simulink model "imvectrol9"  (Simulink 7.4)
settings: Solver=ode45  StartTime=0  StopTime=7  MaxStep=1e-3  RelTol=1e-4  AbsTol=1e-3
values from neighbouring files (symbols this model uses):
  Lm = eval(get(hLm,'String'))    [im3d.m]    (also in IMabc2.m = 4.5; imabcparam.m = 0.0847; IMabcrun0.m = 0.0847; IMabcrun1.m = 0.0847)
  Lr = Lrl+Lm    (= 4.6)    [IMabc2.m]    (also in IMabcf0.m = Lrl+Lm1; IMabcf1.m = Lrl+Lm1; imabcparam.m = 0.0589666666667; IMcur0.m)
  Lrl = eval(get(hLr,'String'))    [im3d.m]    (also in IMabc2.m = 0.1; imabcparam.m = 0.0025; IMabcrun0.m = 0.0025; IMabcrun1.m = 0.0025)
  Ls = Lsl+Lm    (= 4.6)    [IMabc2.m]    (also in IMabcf0.m = Lsl+Lm1; IMabcf1.m = Lsl+Lm1; imabcparam.m = 0.0589666666667; IMcur0.m)
  Lsl = eval(get(hLs,'String'))    [im3d.m]    (also in IMabc2.m = 0.1; imabcparam.m = 0.0025; IMabcrun0.m = 0.0025; IMabcrun1.m = 0.0025)
  Rr = input('Rotor resistance)[default = 2] =')    [Actac.m]    (also in im1phase.m = 0.3; im3d.m = eval(get(hRr,'String')); IMabc2.m = 0.02; imabcparam.m = 0.408)
  Rs = eval(get(hRs,'String'))    [im3d.m]    (also in IMabc2.m = 0.01; imabcparam.m = 0.531; IMabcrun0.m = 0.531; IMabcrun1.m = 0.531)
  wo = 2*pi*freq0    [calc0.m]    (also in IMabc2.m = 376.991118431; imabcparam.m = 376.991118431; IMabcrun0.m = 376.991118431; IMabcrun1.m = 376.991118431)
undefined symbols (not defined in the file or in its folder): fro, Lsp, Tr

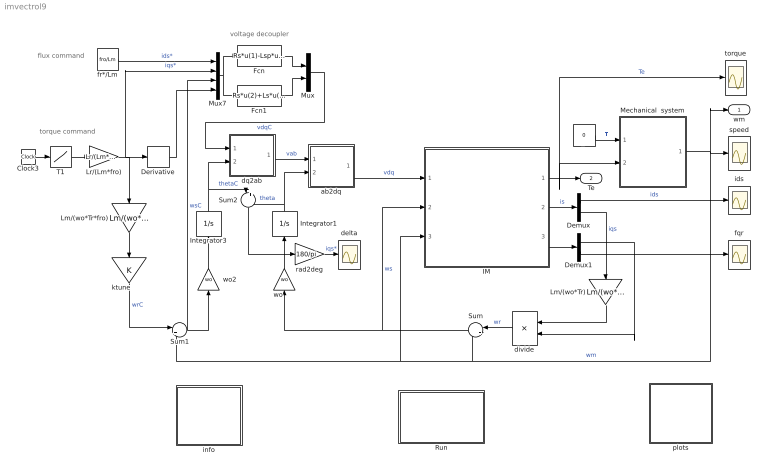
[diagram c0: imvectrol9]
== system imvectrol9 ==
  note: torque command
  note: flux command
  note: voltage decoupler
  Clock3 : Clock
  Demux : Demux  Outputs=2
  Demux1 : Demux  Outputs=2
  Derivative : Derivative
  Fcn : Fcn  Expr=Rs*u(1)-Lsp*u(2)*u(3)
  Fcn1 : Fcn  Expr=Rs*u(2)+Ls*u(1)*u(3)+Lsp*u(4)/wo
  IM : Subsystem
  Integrator1 : Integrator
  Integrator3 : Integrator
  Lm/(wo*Tr) : Gain  Gain=Lm/(wo*Tr)  ParameterDataType=sfix(16)  ParameterScaling=2^0  OutDataType=sfix(16)  OutScaling=2^0
  Lm/(wo*Tr*fro) : Gain  Gain=Lm/(wo*Tr*fro)  ParameterDataType=sfix(16)  ParameterScaling=2^0  OutDataType=sfix(16)  OutScaling=2^0
  Lr/(Lm*fro) : Gain  Gain=Lr/(Lm*fro)  ParameterDataType=sfix(16)  ParameterScaling=2^0  OutDataType=sfix(16)  OutScaling=2^0
  Mechanical  system : Subsystem  mask{H=0.3, Bm=1e-5}
      mask prompts: H "Inertia constant [s]"; Bm "Torque-speed coefficient"
  Mux : Mux  Inputs=2
  Mux7 : Mux
  Run : Subsystem
  Sum : Sum  Inputs=|++  OutDataType=sfix(16)  OutScaling=2^0
  Sum1 : Sum  Inputs=|++  OutDataType=sfix(16)  OutScaling=2^0
  Sum2 : Sum  Inputs=|+-  OutDataType=sfix(16)  OutScaling=2^0
  T1 : Lookup  InputValues=[0 1 1.5 2.5 3.5 4.5 5 8]  Table=[0 0 1 1 -1 -1 0 0]  OutDataType=sfix(16)  OutScaling=2^0
  Tl : Constant  Value=0  OutDataType=sfix(16)  OutScaling=2^0
  ab2dq : Subsystem
  delta : Scope
  divide : Product  Inputs=*/  OutDataType=sfix(16)  OutScaling=2^0
  dq2ab : Subsystem
  fqr : Scope
  fr*/Lm : Constant  Value=fro/Lm  OutDataType=sfix(16)  OutScaling=2^0
  ids : Scope
  info : Subsystem
  ktune : Gain  ParameterDataType=sfix(16)  ParameterScaling=2^0  OutDataType=sfix(16)  OutScaling=2^0
  plots : Subsystem
  rad2deg : Gain  Gain=180/pi  ParameterDataType=sfix(16)  ParameterScaling=2^0  OutDataType=sfix(16)  OutScaling=2^0
  speed : Scope
  torque : Scope
  wo : Gain  Gain=wo  ParameterDataType=sfix(16)  ParameterScaling=2^0  OutDataType=sfix(16)  OutScaling=2^0
  wo2 : Gain  Gain=wo  ParameterDataType=sfix(16)  ParameterScaling=2^0  OutDataType=sfix(16)  OutScaling=2^0
  wm : Outport
  Te : Outport  Port=2
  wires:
  Tl/1 -> Mechanical  system/1(Tl)  "Tl"
  Mechanical  system/1(wm) -> speed/1, Sum/2, IM/3(wm), Sum1/2, wm/1  "wm"
  IM/3(fr) -> Demux1/1
  Demux/2 -> Lm/(wo*Tr)/1  "iqs"
  Sum/1 -> IM/2(Iwk), wo/1  "ws"
  wo/1 -> Integrator1/1
  wo2/1 -> Integrator3/1
  Sum1/1 -> wo2/1, Mux7/3  "wsC"
  IM/1(Te) -> Mechanical  system/2(Te), torque/1, Te/1  "Te"
  Lm/(wo*Tr)/1 -> divide/1
  divide/1 -> Sum/1  "wr"
  dq2ab/1(ab) -> ab2dq/1(ab)  "vab"
  Fcn/1 -> Mux/1
  Mux/1 -> dq2ab/1(dq)  "vdqC"
  Mux7/1 -> Fcn/1, Fcn1/1
  Fcn1/1 -> Mux/2
  fr*/Lm/1 -> Mux7/1  "ids*"
  Lm/(wo*Tr*fro)/1 -> ktune/1
  Lr/(Lm*fro)/1 -> Mux7/2, Lm/(wo*Tr*fro)/1, Derivative/1  "iqs*"
  ktune/1 -> Sum1/1  "wrC"
  Clock3/1 -> T1/1
  T1/1 -> Lr/(Lm*fro)/1
  Derivative/1 -> Mux7/4
  Demux1/2 -> fqr/1
  ab2dq/1(dq) -> IM/1(vs)  "vdq"
  Demux/1 -> ids/1  "ids"
  Demux1/1 -> divide/2
  Integrator3/1 -> dq2ab/2(theta), Sum2/1  "thetaC"
  Integrator1/1 -> ab2dq/2(theta), Sum2/2  "theta"
  IM/2(is) -> Demux/1  "is"
  Sum2/1 -> rad2deg/1
  rad2deg/1 -> delta/1  "iqs*"

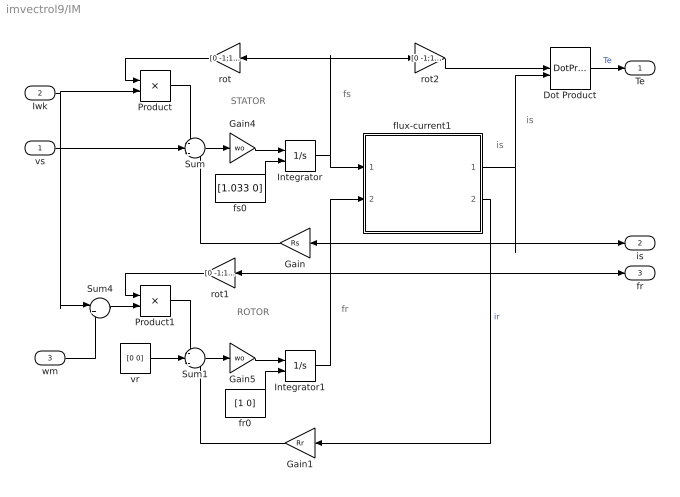
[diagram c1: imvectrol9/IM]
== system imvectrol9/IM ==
  note: ROTOR
  note: STATOR
  note: fs
  note: fr
  note: is
  note: is
  vs : Inport  OutDataType=sfix(16)  OutScaling=2^0
  Iwk : Inport  Port=2  OutDataType=sfix(16)  OutScaling=2^0
  wm : Inport  Port=3  OutDataType=sfix(16)  OutScaling=2^0
  Dot Product : DotProduct  OutDataType=fixdt(1, 16)  OutScaling=2^-10
  Gain : Gain  Gain=Rs  ParameterDataType=sfix(16)  ParameterScaling=2^0  OutDataType=sfix(16)  OutScaling=2^0
  Gain1 : Gain  Gain=Rr  ParameterDataType=sfix(16)  ParameterScaling=2^0  OutDataType=sfix(16)  OutScaling=2^0
  Gain4 : Gain  Gain=wo  ParameterDataType=sfix(16)  ParameterScaling=2^0  OutDataType=sfix(16)  OutScaling=2^0
  Gain5 : Gain  Gain=wo  ParameterDataType=sfix(16)  ParameterScaling=2^0  OutDataType=sfix(16)  OutScaling=2^0
  Integrator : Integrator  InitialConditionSource=external  InitialCondition=[1 0]
  Integrator1 : Integrator  InitialConditionSource=external  InitialCondition=[1 0]
  Product : Product  OutDataType=sfix(16)  OutScaling=2^0
  Product1 : Product  OutDataType=sfix(16)  OutScaling=2^0
  Sum : Sum  Inputs=-+-  OutDataType=sfix(16)  OutScaling=2^0
  Sum1 : Sum  Inputs=-+-  OutDataType=sfix(16)  OutScaling=2^0
  Sum4 : Sum  Inputs=|+-  OutDataType=sfix(16)  OutScaling=2^0
  flux-current1 : Subsystem
  fr0 : Constant  Value=[1 0]  OutDataType=sfix(16)  OutScaling=2^0
  fs0 : Constant  Value=[1.033 0]  OutDataType=sfix(16)  OutScaling=2^0
  rot : Gain  Gain=[0 -1;1 0]  Multiplication=Matrix(K*u)  ParameterDataType=sfix(16)  ParameterScaling=2^0  OutDataType=sfix(16)  OutScaling=2^0
  rot1 : Gain  Gain=[0 -1;1 0]  Multiplication=Matrix(K*u)  ParameterDataType=sfix(16)  ParameterScaling=2^0  OutDataType=sfix(16)  OutScaling=2^0
  rot2 : Gain  Gain=[0 -1;1 0]  Multiplication=Matrix(K*u)  ParameterDataType=sfix(16)  ParameterScaling=2^0  OutDataType=sfix(16)  OutScaling=2^0
  vr : Constant  Value=[0 0]  OutDataType=sfix(16)  OutScaling=2^0
  Te : Outport
  is : Outport  Port=2
  fr : Outport  Port=3
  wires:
  Gain/1 -> Sum/3
  vr/1 -> Sum1/2
  Integrator/1 -> flux-current1/1(fs), rot/1, rot2/1
  Integrator1/1 -> flux-current1/2(fr), rot1/1, fr/1
  Product1/1 -> Sum1/1
  rot1/1 -> Product1/1
  Product/1 -> Sum/1
  rot/1 -> Product/1
  rot2/1 -> Dot Product/1
  Sum4/1 -> Product1/2
  Sum/1 -> Gain4/1
  Gain4/1 -> Integrator/1
  Sum1/1 -> Gain5/1
  Gain5/1 -> Integrator1/1
  Dot Product/1 -> Te/1  "Te"
  vs/1 -> Sum/2
  Iwk/1 -> Product/2, Sum4/1
  wm/1 -> Sum4/2
  flux-current1/1(is) -> Gain/1, is/1, Dot Product/2
  fr0/1 -> Integrator1/2
  fs0/1 -> Integrator/2
  Gain1/1 -> Sum1/3
  flux-current1/2(ir) -> Gain1/1  "ir"

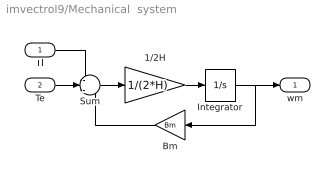
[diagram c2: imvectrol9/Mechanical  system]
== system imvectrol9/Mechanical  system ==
  Tl : Inport  OutDataType=sfix(16)  OutScaling=2^0
  Te : Inport  Port=2  OutDataType=sfix(16)  OutScaling=2^0
  1/2H : Gain  Gain=1/(2*H)  ParameterDataType=sfix(16)  ParameterScaling=2^0  OutDataType=sfix(16)  OutScaling=2^0
  Bm : Gain  Gain=Bm  ParameterDataType=sfix(16)  ParameterScaling=2^0  OutDataType=sfix(16)  OutScaling=2^0
  Integrator : Integrator
  Sum : Sum  Inputs=-+-  OutDataType=sfix(16)  OutScaling=2^0
  wm : Outport
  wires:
  Tl/1 -> Sum/1
  Te/1 -> Sum/2
  Integrator/1 -> wm/1, Bm/1
  Bm/1 -> Sum/3
  Sum/1 -> 1/2H/1
  1/2H/1 -> Integrator/1

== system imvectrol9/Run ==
  note: This demo illustrates the effect of detuning on the vector control of an induction motor
  note: Double click
  note: Edit to modify the parameters

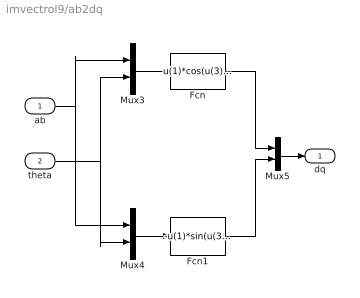
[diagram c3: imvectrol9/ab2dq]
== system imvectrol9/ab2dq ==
  ab : Inport  OutDataType=sfix(16)  OutScaling=2^0
  theta : Inport  Port=2  OutDataType=sfix(16)  OutScaling=2^0
  Fcn : Fcn  Expr=u(1)*cos(u(3))+u(2)*sin(u(3))
  Fcn1 : Fcn  Expr=-u(1)*sin(u(3))+u(2)*cos(u(3))
  Mux3 : Mux  Inputs=2
  Mux4 : Mux  Inputs=2
  Mux5 : Mux  Inputs=2
  dq : Outport
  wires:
  Mux3/1 -> Fcn/1
  Mux4/1 -> Fcn1/1
  Fcn1/1 -> Mux5/2
  Fcn/1 -> Mux5/1
  Mux5/1 -> dq/1
  theta/1 -> Mux4/2, Mux3/2
  ab/1 -> Mux3/1, Mux4/1

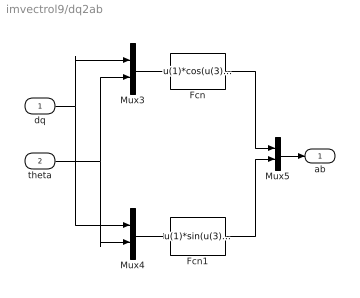
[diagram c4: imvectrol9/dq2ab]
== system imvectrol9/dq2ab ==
  dq : Inport  OutDataType=sfix(16)  OutScaling=2^0
  theta : Inport  Port=2  OutDataType=sfix(16)  OutScaling=2^0
  Fcn : Fcn  Expr=u(1)*cos(u(3))-u(2)*sin(u(3))
  Fcn1 : Fcn  Expr=u(1)*sin(u(3))+u(2)*cos(u(3))
  Mux3 : Mux  Inputs=2
  Mux4 : Mux  Inputs=2
  Mux5 : Mux  Inputs=2
  ab : Outport
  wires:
  dq/1 -> Mux4/1, Mux3/1
  theta/1 -> Mux3/2, Mux4/2
  Mux5/1 -> ab/1
  Fcn/1 -> Mux5/1
  Fcn1/1 -> Mux5/2
  Mux4/1 -> Fcn1/1
  Mux3/1 -> Fcn/1

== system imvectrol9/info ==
  note: Indirect Vector Control of an Induction Motor with Voltage Excitation and Open-Loop Speed Control
  note: Double click the PARAMETERS block to enter the machine parameters . Examine the system dynamic behavior for various values of the ktune factor.

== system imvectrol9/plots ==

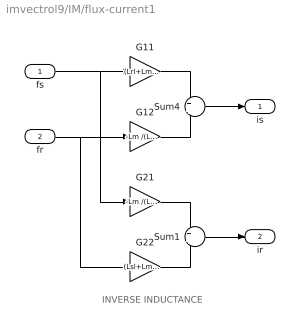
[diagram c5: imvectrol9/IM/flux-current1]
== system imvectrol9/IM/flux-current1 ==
  note: INVERSE INDUCTANCE
  fs : Inport  OutDataType=sfix(16)  OutScaling=2^0
  fr : Inport  Port=2  OutDataType=sfix(16)  OutScaling=2^0
  G11 : Gain  Gain=(Lrl+Lm) /(Lsl*Lrl+Lsl*Lm+Lrl*Lm)  ParameterDataType=sfix(16)  ParameterScaling=2^0  OutDataType=sfix(16)  OutScaling=2^0
  G12 : Gain  Gain=-Lm /(Lsl*Lrl+Lsl*Lm+Lrl*Lm)  ParameterDataType=sfix(16)  ParameterScaling=2^0  OutDataType=sfix(16)  OutScaling=2^0
  G21 : Gain  Gain=-Lm /(Lsl*Lrl+Lsl*Lm+Lrl*Lm)  ParameterDataType=sfix(16)  ParameterScaling=2^0  OutDataType=sfix(16)  OutScaling=2^0
  G22 : Gain  Gain=(Lsl+Lm )/(Lsl*Lrl+Lsl*Lm+Lrl*Lm)  ParameterDataType=sfix(16)  ParameterScaling=2^0  OutDataType=sfix(16)  OutScaling=2^0
  Sum1 : Sum  OutDataType=sfix(16)  OutScaling=2^0
  Sum4 : Sum  OutDataType=sfix(16)  OutScaling=2^0
  is : Outport
  ir : Outport  Port=2
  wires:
  fs/1 -> G11/1, G21/1
  G11/1 -> Sum4/1
  fr/1 -> G12/1, G22/1
  G12/1 -> Sum4/2
  Sum4/1 -> is/1
  G21/1 -> Sum1/1
  G22/1 -> Sum1/2
  Sum1/1 -> ir/1
